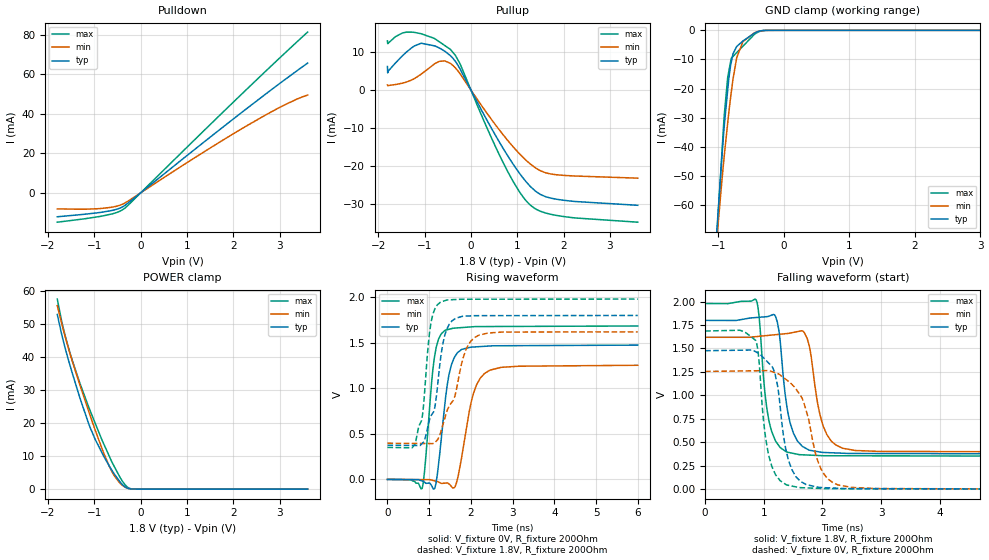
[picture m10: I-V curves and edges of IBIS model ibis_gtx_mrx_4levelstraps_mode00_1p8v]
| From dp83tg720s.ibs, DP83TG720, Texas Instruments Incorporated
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| ibis_gtx_mrx_4levelstraps_mode00_1p8v
[Model]   ibis_gtx_mrx_4levelstraps_mode00_1p8v
Model_type   I/O
Polarity   Non-Inverting
Enable   Active-Low
Vinl = 0.54
Vinh = 1.26
Vmeas = 0.9
Vref = 0.9
Cref = 2pF
Rref = 100000
|   typ   min   max
C_comp   2.49pF   2.45pF   2.54pF
[Voltage Range]   1.8   1.62   1.98
[Temperature Range]   27   150   -40
[Pullup Reference]   1.8   1.62   1.98
[Pulldown Reference]   0   0   0
[Power Clamp Reference]   1.8   1.62   1.98
[GND Clamp Reference]   0   0   0
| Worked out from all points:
|   slope of the pulldown table from 0 to 0.27 V, typ, clamps not added: 52.7 ohm
|   slope of the pullup table from 0 to 0.27 V, typ, clamps not added: 43.2 ohm
|   GND clamp passes 1 mA (typ) near -0.45 V on its own axis
|   POWER clamp passes 1 mA (typ) near -0.36 V on its own axis
|   falling waveform, V_fixture 1.8V, R_fixture 200Ohm: 20-80 % time 183ps typ, 218ps min, 163ps max; typ from 1.8 V to 0.376 V
|   rising waveform, V_fixture 0V, R_fixture 200Ohm: 20-80 % time 234ps typ, 326ps min, 193ps max; typ from 0 V to 1.47 V
|   rising waveform, V_fixture 1.8V, R_fixture 200Ohm: 20-80 % time 329ps typ, 489ps min, 193ps max; typ from 0.376 V to 1.8 V
|   falling waveform, V_fixture 0V, R_fixture 200Ohm: 20-80 % time 219ps typ, 331ps min, 173ps max; typ from 1.48 V to 0 V
[Pulldown]
|   Voltage   I(typ)   I(min)   I(max)
-1.8V     -12.14mA   -8.138mA   -14.87mA
-1.217V   -10.87mA   -8.307mA   -13.16mA
-855mV    -9.881mA   -7.938mA   -11.87mA
-520.2mV  -8.35mA    -6.791mA   -10.01mA
-358.2mV  -6.641mA   -5.371mA   -8.07mA
1.165V    21.93mA    17.72mA    26.86mA
2.25V     41.92mA    33.37mA    51.53mA
3.065V    56.45mA    43.99mA    69.67mA
3.6V      65.57mA    49.42mA    81.25mA
[GND Clamp]
|   Voltage   I(typ)   I(min)   I(max)
-1.8V     -379.6mA   -329.3mA   -423.1mA
-1.017V   -67.63mA   -70.66mA   -69.46mA
-903.6mV  -31.87mA   -42.25mA   -28.2mA
-855mV    -20.54mA   -31.86mA   -16.22mA
-838.8mV  -16.76mA   -28.4mA    -14.23mA
-801mV    -11.03mA   -21.37mA   -9.591mA
-774mV    -8.085mA   -16.75mA   -8.964mA
-714.6mV  -5.501mA   -9.181mA   -7.586mA
-622.8mV  -3.665mA   -3.879mA   -5.456mA
-444.6mV  -924.3uA   -826.8uA   -1.321mA
-255.6mV  -12.26uA   -28.29uA   -12.59uA
3.6V      0A         0A         0A
[Pullup]
|   Voltage   I(typ)   I(min)   I(max)
-1.8V     6.185mA    1.29mA     12.95mA
-1.795V   4.5mA      1.15mA     12.23mA
-1.476V   9.02mA     1.793mA    15.04mA
-1.076V   12.31mA    4.131mA    14.84mA
-682.2mV  11.09mA    7.524mA    12.72mA
-444.6mV  9.078mA    7.03mA     10.73mA
-239.4mV  5.658mA    4.358mA    7.036mA
343.8mV   -7.913mA   -6.086mA   -9.914mA
797.4mV   -17.43mA   -13.36mA   -21.6mA
1.305V    -25.73mA   -19.76mA   -30.62mA
1.845V    -28.84mA   -22.38mA   -33.11mA
3.6V      -30.44mA   -23.28mA   -34.9mA
[POWER Clamp]
|   Voltage   I(typ)   I(min)   I(max)
-1.8V     52.83mA    55.52mA    57.51mA
-1.681V   45.46mA    48.83mA    49.33mA
-1.546V   38.43mA    41.93mA    42.21mA
-1.319V   27.92mA    31.81mA    32.31mA
-1.082V   18.31mA    21.88mA    23.38mA
-979.2mV  14.97mA    17.75mA    19.83mA
-806.4mV  10.17mA    11.18mA    13.94mA
-612mV    5.477mA    5.044mA    7.945mA
-444.6mV  2.163mA    1.755mA    3.504mA
-293.4mV  350.1uA    334.1uA    708uA
-109.8mV  25.24uA    27.21uA    30.53uA
3.6V      0A         0A         0A
[Ramp]
R_load = 200
|   typ   min   max
dV/dt_r   0.884271/2.32054e-10   0.751474/3.22285e-10   1.01019/1.92491e-10
dV/dt_f   0.854139/1.80694e-10   0.733382/2.14764e-10   0.976686/1.62608e-10
[Falling Waveform]
V_fixture = 1.8V
V_fixture_min = 1.62V
V_fixture_max = 1.98V
R_fixture = 200Ohm
C_fixture = 0F
|   Time   V(typ)   V(min)   V(max)
0s        1.799V     1.619V     1.979V
869.7ps   1.83V      1.627V     2.019V
1.085ns   1.843V     1.64V      741.4mV
1.231ns   1.782V     1.649V     486.8mV
1.378ns   951.7mV    1.658V     400.5mV
1.505ns   596.6mV    1.671V     381.1mV
1.691ns   444.6mV    1.669V     365.6mV
2.009ns   391.6mV    679.5mV    356.8mV
2.346ns   383.2mV    436.3mV    356.1mV
6ns       375.8mV    397mV      351.4mV
[Rising Waveform]
V_fixture = 0V
V_fixture_min = 0V
V_fixture_max = 0V
R_fixture = 200Ohm
C_fixture = 0F
|   Time   V(typ)   V(min)   V(max)
0s        113.4uV    256.6uV    67.81uV
829.7ps   -17.42mV   -1.925mV   -100.6mV
887.5ps   -30.22mV   -2.077mV   80.55mV
1.139ns   -90.83mV   -16.93mV   1.372V
1.368ns   789.1mV    -41.31mV   1.632V
1.477ns   1.153V     -50.99mV   1.648V
1.676ns   1.39V      1.06mV     1.663V
2.061ns   1.453V     942.8mV    1.676V
2.453ns   1.464V     1.198V     1.678V
6ns       1.474V     1.253V     1.684V
[Rising Waveform]
V_fixture = 1.8V
V_fixture_min = 1.62V
V_fixture_max = 1.98V
R_fixture = 200Ohm
C_fixture = 0F
|   Time   V(typ)   V(min)   V(max)
0s        375.8mV    397mV      351.4mV
659.3ps   372.1mV    394.7mV    384.5mV
841.1ps   398.2mV    394.1mV    709.3mV
1.044ns   698.6mV    393.4mV    1.72V
1.142ns   808.5mV    407.1mV    1.877V
1.273ns   1.325V     513.5mV    1.946V
1.545ns   1.739V     847.2mV    1.972V
1.872ns   1.792V     1.411V     1.977V
2.177ns   1.797V     1.58V      1.978V
6ns       1.799V     1.619V     1.979V
[Falling Waveform]
|Gnd
V_fixture = 0V
V_fixture_min = 0V
V_fixture_max = 0V
R_fixture = 200Ohm
C_fixture = 0F
|   Time   V(typ)   V(min)   V(max)
0s        1.476V     1.255V     1.686V
861.2ps   1.465V     1.262V     1.587V
907.4ps   1.449V     1.263V     1.441V
1.078ns   1.347V     1.263V     377.1mV
1.234ns   1.107V     1.233V     126.8mV
1.378ns   419.2mV    1.17V      49.17mV
1.624ns   83.38mV    1.001V     16.41mV
1.969ns   17.93mV    224.4mV    7.5mV
2.263ns   9.46mV     45.91mV    5.371mV
6ns       112.5uV    256.9uV    66.75uV
